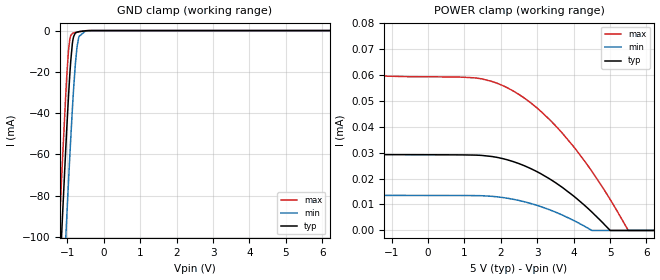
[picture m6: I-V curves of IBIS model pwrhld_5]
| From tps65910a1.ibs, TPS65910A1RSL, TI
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|   pwrhld_5 Model
[Model]   pwrhld_5
Model_type   Input
Vinl = 0.45
Vinh = 1.3
|   typ   min   max
|   (nom PVT)   (fast PVT)   (slow PVT)
C_comp   1.531e-13   1.517e-13   1.557e-13
| Where nom  PVT is Nominal Process, 5V, 27C
|   Fast PVT is Strong Process,  5.5V, -40C
|   Slow PVT is Weak Process,   4.5V, 125C
[Voltage Range]   5   4.5   5.5
|Junction Temperature
[Temperature Range]   27   125   -40
[Power Clamp Reference]   5   4.5   5.5
[GND Clamp Reference]   0   0   0
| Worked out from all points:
|   GND clamp passes 1 mA (typ) near -0.76 V on its own axis
[GND Clamp]
|   Voltage   I(typ)   I(min)   I(max)
-5V       -1.695A    -1.73A     -1.675A
-1.293V   -150.8mA   -194.9mA   -123.3mA
-1.179V   -106.6mA   -150.8mA   -79.11mA
-1.14V    -91.61mA   -135.7mA   -64.21mA
-1.04V    -55.03mA   -98.25mA   -28.94mA
-974mV    -32.92mA   -74.48mA   -10.52mA
-935.5mV  -21.5mA    -61.14mA   -4.275mA
-851mV    -4.664mA   -34.1mA    -1.28mA
-734mV    -748uA     -7.567mA   -718.8uA
-684.5mV  -540.6uA   -2.849mA   -531.9uA
-500mV    -94.11uA   -183.2uA   -66.4uA
10V       0A         0A         0A
[POWER Clamp]
|   Voltage   I(typ)   I(min)   I(max)
-5V       1.209mA    1.229mA    1.686mA
-2.515V   188uA      121.3uA    391.5uA
-2.377V   134.3uA    68.19uA    321uA
-2.22V    77.2uA     23.28uA    242.2uA
-2.055V   33.69uA    13.65uA    161.4uA
-1.873V   29.19uA    13.5uA     81.31uA
-1.75V    29.18uA    13.5uA     59.61uA
1.3V      29.01uA    13.42uA    58.71uA
2.645V    24.92uA    11.06uA    50.96uA
4.05V     12.68uA    3.507uA    31.36uA
5.5V      0A         0A         12.64nA
10V       0A         0A         0A
